FUNCTION_BLOCK FB_SeparatingModule EXTENDS FB_Module
// Module to separate via sensor, barrier and clamp cylinder and axis
VAR_INPUT
		(***** Information about the state and mode of machine *****)
	bExecute					: BOOL;
	bSemiStart					: BOOL;
		(****** Variables to enable / disable diagnosis and temperature mode ******)
	bClampDiag					: BOOL;
	bClampTemp					: BOOL;
	bClampRecord				: BOOL;
	bBarrierDiag				: BOOL;
	bBarrierTemp				: BOOL;
	bBarrierRecord				: BOOL;
		(***** Timer values for clamp and barrier cylinder *****)
	tiTimeOutClamp				: TIME;
	tiTimeOutBarrier			: TIME;
	tiRecordIntervallClamp		: TIME;
	tiRecordIntervallBarrier	: TIME;
	tiBarrierAtWork				: TIME;
		(***** Information about number of boxes being sorted *****)
	iBoxesOnTheWay				: INT;
		(***** Buttons *****)
	bButtonClampToWorkIn		: BOOL;
	bButtonClampToBaseIn		: BOOL;
	bButtonBarrierToWorkIn		: BOOL;
	bButtonBarrierToBaseIn		: BOOL;
END_VAR
VAR_OUTPUT
	bClampToWork				: BOOL;
	bClampAtBase				: BOOL;
	bClampAtWork				: BOOL;
	bBarrierToWork				: BOOL;
	bBarrierAtBase				: BOOL;
	bBarrierAtWork				: BOOL;
	bClampError					: BOOL;
	sClampErrorMsg				: STRING;
	bBarrierError				: BOOL;
	sBarrierErrorMsg			: STRING;
	lrClampTemps				: ARRAY[1..100] OF LREAL;
	lrBarrierTemps				: ARRAY[1..100] OF LREAL;
	bSeparated					: BOOL;
	bButtonClampToWorkOut		: BOOL;
	bButtonClampToBaseOut		: BOOL;
	bButtonBarrierToWorkOut		: BOOL;
	bButtonBarrierToBaseOut		: BOOL;
END_VAR
VAR
(* ================= Function block and interface instances ===================== *)
	
	fbSensor					: FB_SignalHandling;
	
		(* Instances of clamp cylinder function blocks *)
	fbClamp						: FB_Cylinder;					// Without diagnosis and temperature mode
	fbClampDiag					: FB_CylinderDiag;				// With diagnosis of states
	fbClampTemp					: FB_CylinderTemp;				// With temperature mode
	fbClampTempDiag				: FB_CylinderTempDiag;			// With diagnosis of temperature
	fbClampTempRecord			: FB_CylinderTempRecord;		// With record of temperatures
		(* Interface instance of ICylinder for clamp cylinder *)
	iClamp						: ICylinder;
	
			(* Instances of barrier cylinder function blocks *)
	fbBarrier					: FB_Cylinder;					// Without diagnosis and temperature mode
	fbBarrierDiag				: FB_CylinderDiag;				// With diagnosis of states
	fbBarrierTemp				: FB_CylinderTemp;				// With temperature mode
	fbBarrierTempDiag			: FB_CylinderTempDiag;			// With diagnosis of temperature
	fbBarrierTempRecord			: FB_CylinderTempRecord;		// With record of temperatures
		(* Interface instance of ICylinder for barrier cylinder *)
	iBarrier					: ICylinder;
	
				(***** Manual cylinder control *****)
	fbButtonClampToWork			: FB_SignalHandlingIntern;		// To move manually clamp cylinder to work position
	fbButtonClampToBase			: FB_SignalHandlingIntern;		// To move manually clamp cylinder to base position
	fbButtonBarrierToWork		: FB_SignalHandlingIntern;		// To move manually barrier cylinder to work position
	fbButtonBarrierToBase		: FB_SignalHandlingIntern;		// To move manually barrier cylinder to base position
	
(* ========================== COMMON VARIABLES =============================== *)	
	tonBarrierAtWork			: TON;							// Timer for opening barrier in AUTOMATIC mode
END_VAR

// =========================================================
;
// =========================================================

METHOD PUBLIC M_Automatic
VAR_INPUT
END_VAR
// =========================================================
	// Noticing work position of barrier cylinder	

tonBarrierAtWork( PT := tiBarrierAtWork );

// =========================================================
	// Control of main axis

IF NOT bHalt THEN
	fbAxis.M_MoveFw();
ELSIF NOT bHaltDone THEN
	M_Stop();
ELSE
	bHalt := FALSE;
	M_Stop();
END_IF

// =========================================================
	// Process of separating boxes
	
CASE iState OF
	0:	// Init
		iBarrier.M_MoveToBase();					(***** Calling method of FB via interface *****)
		IF iBarrier.P_AtBasePos AND bExecute THEN	(***** Accessing property of FB via interface *****)
			iState := 1;
		END_IF
		
// =========================================================
	1: // Start
		IF fbSensor.bOut AND fbAxis.bMoves THEN
			iState := 2;
		ELSIF NOT iClamp.P_AtWorkPos THEN			(***** Accessing property of FB via interface instance *****)
			iClamp.M_MoveToWork();					(***** Calling method of FB via interface instance *****)
		END_IF
		
// =========================================================
	2: // Closing clamp
		iClamp.M_MoveToBase();						(***** Calling method of FB via interface instance *****)
		IF iClamp.P_AtBasePos THEN					(***** Accessing property of FB via interface instance *****)
			bSeparated := TRUE;
			iState := 3;
		END_IF
		
// =========================================================
	3: // Opening barrier
		iBarrier.M_MoveToWork();					(***** Calling method of FB via interface *****)
		
		IF iBarrier.P_AtWorkPos THEN				(***** Accessing property of FB via interface *****)
			tonBarrierAtWork( IN := TRUE );
		END_IF
		
		IF tonBarrierAtWork.Q THEN
			tonBarrierAtWork( IN := FALSE );
			iState := 4;
		END_IF
		
// =========================================================
	4:	// Closing barrier
		iBarrier.M_MoveToBase();					(***** Calling method of FB via interface *****)
		IF iBarrier.P_AtBasePos THEN				(***** Accessing property of FB via interface *****)
			bSeparated := FALSE;
			iState := 5;
		END_IF
		
// =========================================================
	5:	// Opening clamp
		iClamp.M_MoveToWork();						(***** Calling method of FB via interface instance *****)
		IF iClamp.P_AtWorkPos THEN					(***** Accessing property of FB via interface instance *****)
			iState := 0;
		END_IF
END_CASE

// =========================================================
END_METHOD

METHOD PUBLIC M_CylinderOptions
VAR_INPUT
END_VAR
// =========================================================
		// Selecting clamp cylinder

// Checking variables to enable / disable diagnosis and temperature mode
IF bClampDiag THEN
	IF bClampTemp THEN
		
	(* ============== FB with diagnosis and temperature mode ============== *)
		bClampError := fbClampTempDiag.bError;		// Assigning global output variable to output variable of selected FB
		sClampErrorMsg := fbClampTempDiag.sErrorMsg;
		iClamp := fbClampTempDiag;					// Assigning desired FB instance to interface instance
	
	ELSE
	
	(* ============== FB with diagnosis and without temperature mode ============== *)
		fbClampDiag.tiTimeOut := tiTimeOutClamp;	// Setting special data for selected FB
		bClampError := fbClampDiag.bError;			// Assigning global output variable to output variable of selected FB
		sClampErrorMsg := fbClampDiag.sErrorMsg;
		iClamp := fbClampDiag;						// Assigning desired FB instance to interface instance
	END_IF
ELSE
	bClampError := FALSE;
	sClampErrorMsg := '';
	
	IF bClampTemp THEN
		IF bClampRecord THEN
			fbClampTempRecord.tiIntervalTime := tiRecordIntervallClamp;	// Time of record interval
			fbClampTempRecord.bRecordStart := bComprAirEnabled;			// Recording if compressed air is set
			fbClampTempRecord.M_Record();								// Calling method of function block FB_CylinderTempRecord
			lrClampTemps := fbClampTempRecord.lrTemps;					// Saving output variable
			iClamp := fbClampTempRecord;
		ELSE
			(* ============== FB without diagnosis and with temperature mode ============== *)
			iClamp := fbClampTemp; 						// Assigning desired FB instance to interface instance
		END_IF
	ELSE
	
	(* ============== FB without diagnosis and temperature mode ============== *)
		iClamp := fbClamp;							// Assigning desired FB instance to interface instance						
	END_IF	
END_IF
									
// =========================================================
// =========================================================
			(**** Selecting barrier cylinder ****)

// Checking variables to enable / disable diagnosis and temperature mode
IF bBarrierDiag THEN
	IF bBarrierTemp THEN
		
	(* ============== FB with diagnosis and temperature mode ============== *)
		bBarrierError := fbBarrierTempDiag.bError;		// Assigning global output variable to output variable of selected FB
		sBarrierErrorMsg := fbBarrierTempDiag.sErrorMsg;
		iBarrier := fbBarrierTempDiag;					// Assigning desired FB instance to interface instance
	
	ELSE
	
	(* ============== FB with diagnosis and without temperature mode ============== *)
		fbBarrierDiag.tiTimeOut := tiTimeOutBarrier;	// Setting special data for selected FB
		bBarrierError := fbBarrierDiag.bError;			// Assigning global output variable to output variable of selected FB
		sBarrierErrorMsg := fbBarrierDiag.sErrorMsg;
		iBarrier := fbBarrierDiag;						// Assigning desired FB instance to interface instance
	END_IF
ELSE
	bBarrierError := FALSE;
	sBarrierErrorMsg := '';
	
	IF bBarrierTemp THEN
		IF bBarrierRecord THEN
			fbBarrierTempRecord.tiIntervalTime := tiRecordIntervallBarrier;// Time of record interval
			fbBarrierTempRecord.bRecordStart := bComprAirEnabled;			// Recording if compressed air is set
			fbBarrierTempRecord.M_Record();									// Calling method of function block FB_CylinderTempRecord
			lrBarrierTemps := fbBarrierTempRecord.lrTemps;					// Saving output variable
			iBarrier := fbBarrierTempRecord;
		ELSE
			(* ============== FB without diagnosis and with temperature mode ============== *)
			iBarrier := fbBarrierTemp; 						// Assigning desired FB instance to interface instance
		END_IF
	ELSE
	
	(* ============== FB without diagnosis and temperature mode ============== *)
		iBarrier := fbBarrier;							// Assigning desired FB instance to interface instance						
	END_IF	
END_IF
									
// =========================================================
END_METHOD

METHOD PUBLIC M_Enable
VAR_INPUT
END_VAR
// =========================================================
		// Calling method M_Enable of base class FB_Module via 'SUPER^.'
		
SUPER^.M_Enable();

// =========================================================
		// Sensor control
		
fbSensor.bEnable := bSensorEnable;

// =========================================================
		// Cylinder control
		
fbButtonClampToWork.bEnable := bManualCylinderEnable
								AND NOT iClamp.P_AtWorkPos;		(*** Accessing property of FB via interface instance ***)
fbButtonClampToBase.bInput := NOT fbButtonClampToWork.bInput;
fbButtonClampToBase.bEnable := bManualCylinderEnable
								AND NOT iClamp.P_AtBasePos;		(*** Accessing property of FB via interface instance ***)

fbButtonBarrierToWork.bEnable := bManualCylinderEnable
								AND NOT iBarrier.P_AtWorkPos;	(*** Accessing property of FB via interface instance ***)
fbButtonBarrierToBase.bInput := NOT fbButtonBarrierToWork.bInput;
fbButtonBarrierToBase.bEnable := bManualCylinderEnable
								AND NOT iBarrier.P_AtBasePos;	(*** Accessing property of FB via interface instance ***)

// =========================================================
END_METHOD

METHOD PUBLIC M_Maintenance
VAR_INPUT
END_VAR
// =========================================================
	// Calling own method M_Manual of this class FB_SeparatingModule via 'THIS^.'
		
THIS^.M_Manual();				

// =========================================================
END_METHOD

METHOD PUBLIC M_Manual
VAR_INPUT
END_VAR
// =========================================================
	// Calling method M_Manual of base class FB_Module via 'SUPER^.'
		
SUPER^.M_Manual();							

// =========================================================
	// Manual cylinder control
	
IF fbButtonClampToWork.bOut THEN
	iClamp.M_MoveToWork();					(**** Calling method of FB via interface instance ****)
ELSIF fbButtonClampToBase.bOut THEN
	iClamp.M_MoveToBase();					(**** Calling method of FB via interface instance ****)
END_IF

IF fbButtonBarrierToWork.bOut THEN
	iBarrier.M_MoveToWork();				(**** Calling method of FB via interface instance ****)
ELSIF fbButtonBarrierToBase.bOut THEN
	iBarrier.M_MoveToBase();				(**** Calling method of FB via interface instance ****)
END_IF

// =========================================================
END_METHOD

METHOD PUBLIC M_Reset
VAR_INPUT
END_VAR
// =========================================================
		// Resetting cylinder and axis
		
rtrigResetStart( CLK := bReset );

IF rtrigResetStart.Q THEN
	bSeparated := FALSE;
	tonBarrierAtWork( IN := FALSE );
	iClamp.M_Reset();					(**** Calling method of FB via interface ****)
	iBarrier.M_Reset();					(**** Calling method of FB via interface ****)
END_IF

// =========================================================
		// Calling method of base class
		
SUPER^.M_Reset();						// Calling method M_Reset of base class FB_Module via 'SUPER^.'

// =========================================================
END_METHOD

METHOD PUBLIC M_Semiautomatic
VAR_INPUT
END_VAR
// =========================================================
	// Noticing work position of barrier cylinder	

tonBarrierAtWork( PT := tiBarrierAtWork );

// =========================================================
	// Control of main axis

IF iBoxesOnTheWay = 0 AND iState = 0 THEN
	bHalt := TRUE;
	M_Stop();
END_IF

IF bHalt THEN
	IF bHaltDone THEN
		bHalt := FALSE;
	END_IF
	M_Stop();
ELSE
	fbAxis.M_MoveFw();
END_IF

// =========================================================
	// Process of separating boxes
	
CASE iState OF
	0:	// Init
		iBarrier.M_MoveToBase();					(***** Calling method of FB via interface *****)
		IF iBarrier.P_AtBasePos						(***** Accessing property of FB via interface *****)
			AND bExecute AND bSemiStart THEN
				iState := 1;
		END_IF
		
// =========================================================
	1: // Start
		IF fbSensor.bOut THEN
			iState := 2;
		ELSE
			IF NOT iClamp.P_AtWorkPos THEN			(***** Accessing property of FB via interface instance *****)
				iClamp.M_MoveToWork();				(***** Calling method of FB via interface instance *****)
			END_IF
			fbAxis.M_MoveFw();
		END_IF
		
// =========================================================
	2: // Closing clamp
		iClamp.M_MoveToBase();						(***** Calling method of FB via interface instance *****)
		IF iClamp.P_AtBasePos THEN					(***** Accessing property of FB via interface instance *****)
			bSeparated := TRUE;
			iState := 3;
		END_IF
		
// =========================================================
	3: // Opening barrier
		iBarrier.M_MoveToWork();					(***** Calling method of FB via interface *****)
		
		IF iBarrier.P_AtWorkPos THEN				(***** Accessing property of FB via interface *****)
			tonBarrierAtWork( IN := TRUE );
		END_IF
		
		IF tonBarrierAtWork.Q THEN
			tonBarrierAtWork( IN := FALSE );
			iState := 4;
		END_IF
		
// =========================================================
	4:	// Closing barrier
		iBarrier.M_MoveToBase();					(***** Calling method of FB via interface *****)
		IF iBarrier.P_AtBasePos THEN				(***** Accessing property of FB via interface *****)
			bSeparated := FALSE;
			iState := 5;
		END_IF
		
// =========================================================
	5:	// Opening clamp
		iClamp.M_MoveToWork();						(***** Calling method of FB via interface instance *****)
		IF iClamp.P_AtWorkPos THEN					(***** Accessing property of FB via interface instance *****)
			iState := 0;
		END_IF
END_CASE

// =========================================================
END_METHOD

METHOD PUBLIC M_SetOutput
VAR_INPUT
END_VAR
// =========================================================
		// Calling method M_SetOutput of base class FB_Module via 'SUPER^.'
		
SUPER^.M_SetOutput();						

// =========================================================
		// Sensor
		
fbSensor.M_SetOutput();

// =========================================================
		// Cylinder buttons
		
fbButtonClampToWork.M_SetOutput();
fbButtonClampToBase.M_SetOutput();
fbButtonBarrierToWork.M_SetOutput();
fbButtonBarrierToBase.M_SetOutput();

// =========================================================
		// Output variables for cylinders
		
bClampToWork := iClamp.P_ToWork;			// Assigning global output variable to property of selected FB
											// Accessing property of selected FB via interface instance
bClampAtWork := iClamp.P_AtWorkPos;
bClampAtBase := iClamp.P_AtBasePos;
		
bBarrierToWork := iBarrier.P_ToWork;		// Assigning global output variable to property of selected FB
											// Accessing property of selected FB via interface instance
bBarrierAtWork := iBarrier.P_AtWorkPos;
bBarrierAtBase := iBarrier.P_AtBasePos;

// =========================================================
		// Buttons

fbButtonClampToWork.bInput := bButtonClampToWorkIn;
fbButtonClampToBase.bInput := bButtonClampToBaseIn;
fbButtonBarrierToWork.bInput := bButtonBarrierToWorkIn;
fbButtonBarrierToBase.bInput := bButtonBarrierToBaseIn;
bButtonClampToWorkOut := fbButtonClampToWork.bOut;
bButtonClampToBaseOut := fbButtonClampToBase.bOut;
bButtonBarrierToWorkOut := fbButtonBarrierToWork.bOut;
bButtonBarrierToBaseOut := fbButtonBarrierToBase.bOut;

// =========================================================
END_METHOD

END_FUNCTION_BLOCK
